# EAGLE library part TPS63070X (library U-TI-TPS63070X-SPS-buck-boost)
TPS63070 2-V to 16-V Buck-Boost Converter With 3.6-A Switch Current
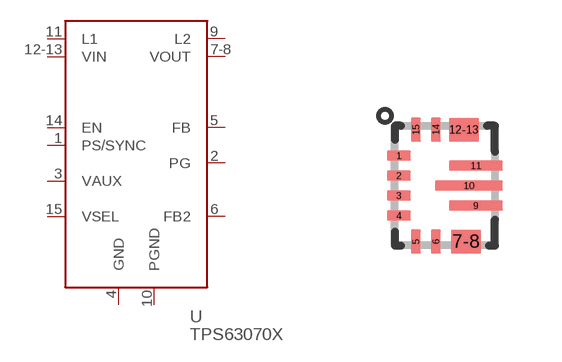
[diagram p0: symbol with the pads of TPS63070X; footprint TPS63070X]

Designator prefix U

## TPS63070X  [TPS63070X]
1  PS/SYNC  in
2  PG  oc
3  VAUX  out
4  GND  pwr
5  FB  pas
6  FB2  pas
7-8  VOUT  pwr
9  L2  pas
10  PGND  pwr
11  L1  pas
12-13  VIN  pwr
14  EN  in
15  VSEL  in

## Footprint TPS63070X (pad centres in mm)
smd 0.6 x 0.25: 1 -1.15,0.75; 2 -1.15,0.25; 3 -1.15,-0.25; 4 -1.15,-0.75
smd 0.25 x 0.6: 5 -0.725,-1.4; 6 -0.225,-1.4; 14 -0.225,1.4; 15 -0.725,1.4
smd 0.75 x 0.6: 7-8 0.525,-1.4; 12-13 0.475,1.4
smd 1.35 x 0.25: 9 0.775,-0.5; 11 0.775,0.5
smd 1.7 x 0.25: 10 0.6,0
